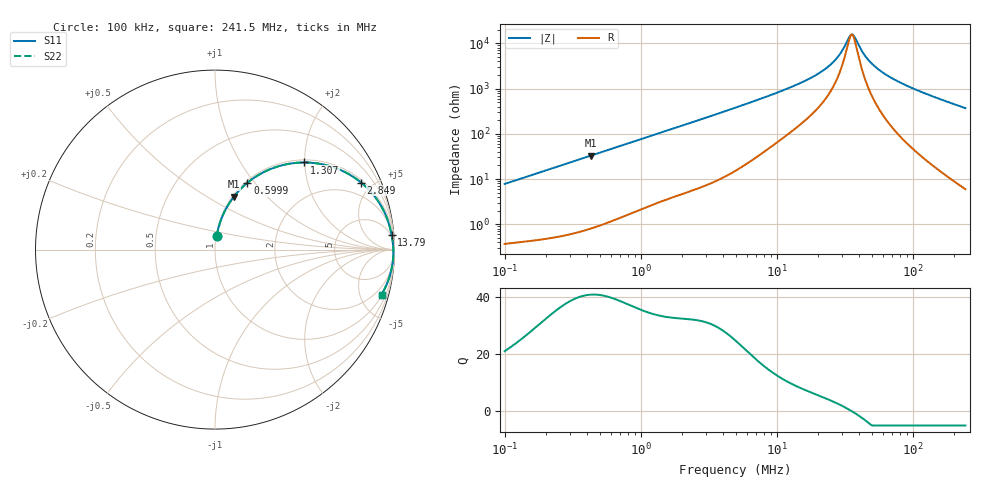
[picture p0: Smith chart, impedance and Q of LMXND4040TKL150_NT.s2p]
! LMXND4040TKL150_NT  S-PARAMETER MODEL  ( Standard Model )
! Model Generated by TAIYO YUDEN Corporation (https://www.yuden.co.jp/en/)
! Version 1.0
! TAIYO YUDEN Control No. 20251120
! Copyright(c) 2025 TAIYO YUDEN CO.,LTD. All Rights Reserved.
! Product Description (link to TY-COMPAS)
! https://ds.yuden.co.jp/TYCOMPAS/or/detail?pn=LMXND4040TKL150MNT&u=M
! Products Name : Inductors
! Characteristics :
!  Inductance : 15 [uH] , SRF(min) : 18 [MHz] , DC Resistance(max) : 0.252 [Ohm]
!  Rated Current : Saturation  1100 [mA] , Temp Rise  1300 [mA] (40 [degC])
!  Case Size : 4.0 x 4.0 / 0.157 x 0.157 [mm/inch] , Thickness : 1.8 / 0.071 [mm/inch]
!  (Conditions: Temperature = 25 [degC] , DC Bias Current = 0 [A])
! External Node Assignments :
!  1  o---GGG---o  2
! GND o---------o GND
! Frequency Range : 0.1MHz  -  241.513628MHz  [ 402 STEP ]
# MHz S RI R 50
! Freq[MHz].  S11 Real  S11 Imag  S21 Real  S21 Imag  S12 Real  S12 Imag  S22 Real  S22 Imag
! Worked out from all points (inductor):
!   401 points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, 100 kHz to 241.5 MHz, reference 50 ohm
!   read as one part in series: L = 12.4 uH near 104 kHz
!   highest Q = 40.9 at 430.8 kHz (marker M1), where L = 12.2 uH
!   self-resonance near 35.13 MHz
!   S11 on the Smith chart (normalised r, x): 100 kHz: 1.01, +0.16; 599.9 kHz: 1.02, +0.92; 1.307 MHz: 1.06, +1.98; 2.849 MHz: 1.14, +4.30; 13.79 MHz: 4, +24; 241.5 MHz: 1.12, -7.38
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0.1  0.00966 0.0769  0.9903 -0.0769  0.9903 -0.0769  0.00966 0.0769
0.368674  0.0801 0.2593  0.9199 -0.2593  0.9199 -0.2593  0.0801 0.2593
0.430826  0.1048 0.2943  0.8952 -0.2943  0.8952 -0.2943  0.1048 0.2943
0.599897  0.1809 0.3726  0.8191 -0.3726  0.8191 -0.3726  0.1809 0.3726
1.307286  0.4964 0.4854  0.5036 -0.4854  0.5036 -0.4854  0.4964 0.4854
1.359207  0.515 0.4851  0.485 -0.4851  0.485 -0.4851  0.515 0.4851
2.848819  0.8144 0.3733  0.1856 -0.3733  0.1856 -0.3733  0.8144 0.3733
4.914404  0.9252 0.2438  0.0748 -0.2438  0.0748 -0.2438  0.9252 0.2438
13.79465  0.9841 0.0808  0.0159 -0.0808  0.0159 -0.0808  0.9841 0.0808
18.11814  0.9884 0.0544  0.0116 -0.0544  0.0116 -0.0544  0.9884 0.0544
22.44628  0.9908 0.036  0.00918 -0.036  0.00918 -0.036  0.9908 0.036
26.2303  0.9921 0.0234  0.00787 -0.0234  0.00787 -0.0234  0.9921 0.0234
29.48135  0.9929 0.0143  0.00712 -0.0143  0.00712 -0.0143  0.9929 0.0143
33.78694  0.9935 0.00363  0.00648 -0.00363  0.00648 -0.00363  0.9935 0.00363
35.81962  0.9937 -0.000938  0.00629 0.000938  0.00629 0.000938  0.9937 -0.000938
37.24223  0.9938 -0.00399  0.00619 0.00399  0.00619 0.00399  0.9938 -0.00399
41.85813  0.994 -0.0133  0.00603 0.0133  0.00603 0.0133  0.994 -0.0133
47.04613  0.9939 -0.0228  0.00609 0.0228  0.00609 0.0228  0.9939 -0.0228
54.97721  0.9934 -0.0361  0.00656 0.0361  0.00656 0.0361  0.9934 -0.0361
66.79689  0.9921 -0.054  0.00787 0.054  0.00787 0.054  0.9921 -0.054
113.0069  0.9823 -0.114  0.0177 0.114  0.0177 0.114  0.9823 -0.114
241.5136  0.928 -0.2504  0.072 0.2504  0.072 0.2504  0.928 -0.2504
